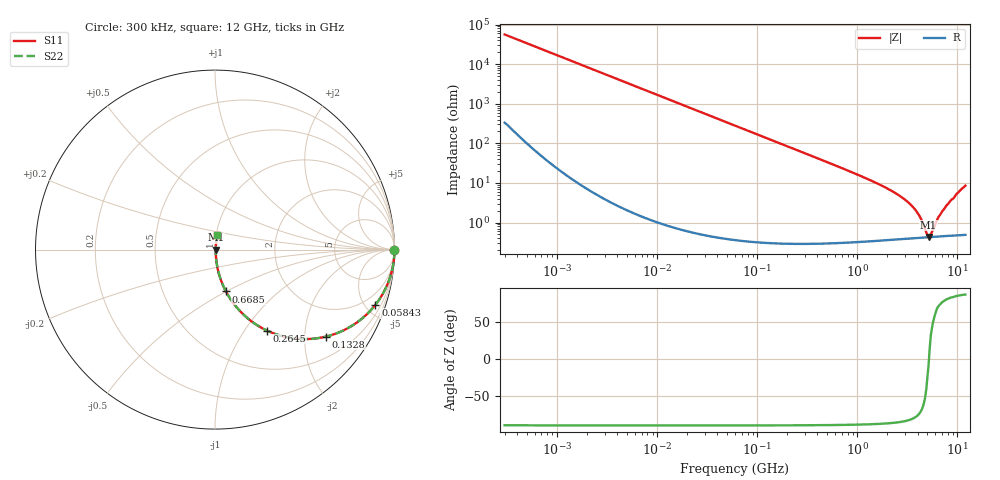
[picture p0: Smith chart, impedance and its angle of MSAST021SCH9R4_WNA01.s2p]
! MSAST021SCH9R4_WNA01  S-PARAMETER MODEL  ( General Type )
! Model Generated by TAIYO YUDEN Corporation (http://www.ty-top.com)
! Version 2.0
! TAIYO YUDEN Control No. 181101
! Copyright(c) 2015 TAIYO YUDEN CO.,LTD. All Rights Reserved.
! Product Description (link to TY-COMPAS)
! https://ds.yuden.co.jp/TYCOMPAS/or/detail?pn=MSAST021SCH9R4CWNA01&u=M
! Products Name : Multilayer Ceramic Capacitors
! Characteristics :
!  Capacitance : 9.4 pF , Rated Voltage : 25V , TCC : CH / C0H
!  Case Size : 0.25 x 0.125 / 0.0098 x 0.0049 [mm/inch] , Thickness : 0.125 / 0.0049 [mm/inch]
!  (Conditions: Temperature = 25 degC , DC Bias Current/Voltage = 0A / 0V)
! External Node Assignments :
!  1  o---| |---o  2
! GND o---------o GND
! Frequency Range : 0.3MHz  -  12000MHz  [ 401 STEP ]
# MHz S RI R 50
! Freq[MHz].  S11 Real  S11 Imag  S21 Real  S21 Imag  S12 Real  S12 Imag  S22 Real  S22 Imag
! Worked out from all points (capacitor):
!   401 points, 300 kHz to 12 GHz, reference 50 ohm
!   read as one part in series: C = 9.4 pF near 316.3 kHz
!   lowest |Z| = 432 mohm at 5.141 GHz (marker M1)
!   series resonance near 5.196 GHz, so ESL is about 100 pH
!   S11 on the Smith chart (normalised r, x): 300 kHz: open; 58.43 MHz: 1.01, -5.79; 132.8 MHz: 1.01, -2.55; 264.5 MHz: 1.01, -1.28; 668.5 MHz: 1.01, -0.50; 12 GHz: 1.01, +0.17
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0.3  1 -0.00177  1.36e-05 0.00177  1.36e-05 0.00177  1 -0.00177
1.769972  0.9999 -0.0105  0.000119 0.0105  0.000119 0.0105  0.9999 -0.0105
10.44266  0.9962 -0.0614  0.00383 0.0614  0.00383 0.0614  0.9962 -0.0614
25.70316  0.9774 -0.1484  0.0226 0.1484  0.0226 0.1484  0.9774 -0.1484
58.43137  0.8932 -0.3082  0.1068 0.3082  0.1068 0.3082  0.8932 -0.3082
60  0.8881 -0.3146  0.1119 0.3146  0.1119 0.3146  0.8881 -0.3146
89.27472  0.782 -0.4121  0.218 0.4121  0.218 0.4121  0.782 -0.4121
132.8329  0.6184 -0.4846  0.3816 0.4846  0.3816 0.4846  0.6184 -0.4846
264.5085  0.2904 -0.4517  0.7096 0.4517  0.7096 0.4517  0.2904 -0.4517
353.9943  0.1862 -0.3863  0.8138 0.3863  0.8138 0.3863  0.1862 -0.3863
668.5285  0.0609 -0.2331  0.9391 0.2331  0.9391 0.2331  0.0609 -0.2331
2088.533  0.00813 -0.067  0.9919 0.067  0.9919 0.067  0.00813 -0.067
2870.14  0.00546 -0.0404  0.9945 0.0404  0.9945 0.0404  0.00546 -0.0404
3642.919  0.00453 -0.0231  0.9955 0.0231  0.9955 0.0231  0.00453 -0.0231
4158.869  0.00429 -0.0142  0.9957 0.0142  0.9957 0.0142  0.00429 -0.0142
4875.354  0.00422 -0.00372  0.9958 0.00372  0.9958 0.00372  0.00422 -0.00372
5140.631  0.00425 -0.00069  0.9958 0.00069  0.9958 0.00069  0.00425 -0.00069
5420.343  0.00429 0.00267  0.9957 -0.00267  0.9957 -0.00267  0.00429 0.00267
6524.734  0.0046 0.0134  0.9954 -0.0134  0.9954 -0.0134  0.0046 0.0134
7448.838  0.00502 0.0223  0.995 -0.0223  0.995 -0.0223  0.00502 0.0223
10236.47  0.00808 0.0575  0.9919 -0.0575  0.9919 -0.0575  0.00808 0.0575
12000  0.0119 0.0836  0.9881 -0.0836  0.9881 -0.0836  0.0119 0.0836
